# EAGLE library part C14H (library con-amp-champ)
CONNECTOR
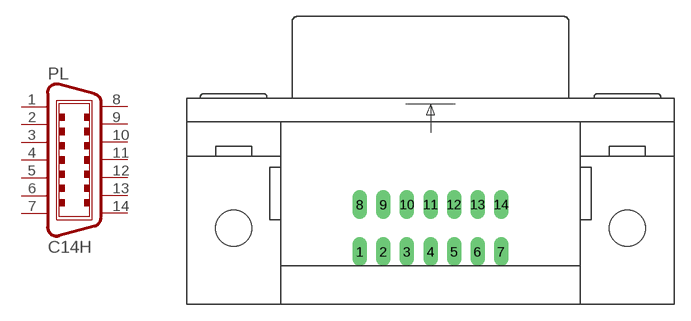
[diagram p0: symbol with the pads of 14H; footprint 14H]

Designator prefix PL

## C14H (OC_FARNELL: unknown; OC_NEWARK: unknown)  [14H]
1  1  pas
2  2  pas
3  3  pas
4  4  pas
5  5  pas
6  6  pas
7  7  pas
8  8  pas
9  9  pas
10  10  pas
11  11  pas
12  12  pas
13  13  pas
14  14  pas

## Footprint 14H (pad centres in mm)
CONNECTOR horizontal with mounting hole
drill 0.813 long: 1 -6.477,-2.159; 2 -4.318,-2.159; 3 -2.159,-2.159; 4 0,-2.159; 5 2.159,-2.159; 6 4.318,-2.159; 7 6.477,-2.159; 8 -6.477,2.159; 9 -4.318,2.159; 10 -2.159,2.159; 11 0,2.159; 12 2.159,2.159; 13 4.318,2.159; 14 6.477,2.159
hole 3.302 at -18.059,0
hole 3.302 at 18.059,0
